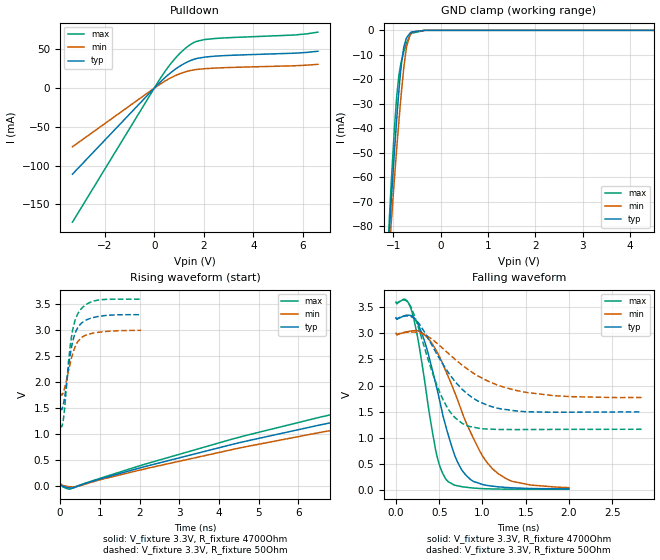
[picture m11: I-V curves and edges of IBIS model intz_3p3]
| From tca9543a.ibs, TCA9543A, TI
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|   intz_3p3 Model
[Model]   intz_3p3
Model_type   Open_drain
Polarity   Non-Inverting
Vmeas = 1.65
Vref = 3.3
Cref = 100pF
Rref = 4700
|   typ   min   max
|   (nom PVT)   (fast PVT)   (slow PVT)
C_comp   1.585e-12   1.479e-12   1.813e-12
| Where nom  PVT is Nominal Process, 3.3V, 27C
|   Fast PVT is Strong Process,  3.6V, -40C
|   Slow PVT is Weak Process,   3V, 85C
[Voltage Range]   3.3   3   3.6
|Junction Temperature
[Temperature Range]   27   85   -40
[Pullup Reference]   3.3   3   3.6
[Pulldown Reference]   0   0   0
[Power Clamp Reference]   3.3   3   3.6
[GND Clamp Reference]   0   0   0
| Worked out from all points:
|   slope of the pulldown table from 0 to 0.495 V, typ, clamps not added: 32.1 ohm
|   GND clamp passes 1 mA (typ) near -0.64 V on its own axis
|   falling waveform, V_fixture 3.3V, R_fixture 4700Ohm: 20-80 % time 309ps typ, 464ps min, 208ps max; typ from 3.3 V to 0.019 V
|   rising waveform, V_fixture 3.3V, R_fixture 4700Ohm: 20-80 % time 18ns typ, 18.9ns min, 17.1ns max; typ from 0.02 V to 3.3 V
|   falling waveform, V_fixture 3.3V, R_fixture 50Ohm: 20-80 % time 455ps typ, 651ps min, 310ps max; typ from 3.3 V to 1.5 V
|   rising waveform, V_fixture 3.3V, R_fixture 50Ohm: 20-80 % time 237ps typ, 266ps min, 218ps max; typ from 1.5 V to 3.3 V
[Pulldown]
|   Voltage   I(typ)   I(min)   I(max)
-3.3V     -111mA     -75.61mA   -172.9mA
243mV     7.977mA    5.352mA    12.58mA
558mV     17.19mA    11.45mA    27.09mA
843.6mV   24.36mA    16.07mA    38.41mA
1.32V     33.59mA    21.66mA    53.11mA
1.647V    37.69mA    23.83mA    59.61mA
2.052V    40.16mA    25.17mA    62.81mA
3.231V    42.56mA    26.86mA    65.44mA
5.642V    45.12mA    28.87mA    68.56mA
6.6V      47.62mA    30.78mA    72.34mA
[GND Clamp]
|   Voltage   I(typ)   I(min)   I(max)
-3.3V     -900.9mA   -814.7mA   -1.047A
-1.169V   -109.9mA   -114.6mA   -110.1mA
-1.047V   -71.3mA    -80.31mA   -64.43mA
-974.4mV  -49.75mA   -60.85mA   -40.2mA
-924mV    -35.82mA   -47.94mA   -26.61mA
-880.8mV  -24.97mA   -37.42mA   -18.62mA
-823.2mV  -13.15mA   -24.49mA   -12.34mA
-775.5mV  -6.819mA   -15.22mA   -8.668mA
-717mV    -3.044mA   -6.672mA   -5.061mA
-612mV    -674.2uA   -730.5uA   -1.179mA
-330mV    -1.399uA   -1.345uA   -1.097uA
6.6V      0A         0A         0A
[POWER Clamp]
|   Voltage   I(typ)   I(min)   I(max)
-3.3V     0A         0A         0A
-3.243V   0A         0A         0A
6.6V      0A         0A         0A
[Ramp]
R_load = 4700
|   typ   min   max
dV/dt_r   1.96775/1.80168e-08   1.7835/1.8882e-08   2.15152/1.71709e-08
dV/dt_f   1.96775/3.0818e-10   1.7835/4.67542e-10   2.15152/2.07559e-10
[Falling Waveform]
V_fixture = 3.3V
V_fixture_min = 3V
V_fixture_max = 3.6V
R_fixture = 4700Ohm
|   Time   V(typ)   V(min)   V(max)
0s        3.3V       3V         3.6V
110ps     3.345V     3.024V     3.65V
190ps     3.329V     3.049V     3.383V
320ps     2.904V     2.987V     2.218V
460ps     2.036V     2.69V      750.4mV
590ps     1.137V     2.226V     179.2mV
790ps     317.7mV    1.373V     53.4mV
1.12ns    69.76mV    397.3mV    16.29mV
1.35ns    37.45mV    160.9mV    12.52mV
2ns       18.86mV    41.74mV    14mV
[Rising Waveform]
V_fixture = 3.3V
V_fixture_min = 3V
V_fixture_max = 3.6V
R_fixture = 4700Ohm
|   Time   V(typ)   V(min)   V(max)
0s        20.41mV    27.49mV    14.13mV
260ps     -38.28mV   -16.59mV   -57.82mV
2.12ns    371.6mV    327.3mV    417mV
6.54ns    1.176V     1.032V     1.325V
11.63ns   1.854V     1.634V     2.08V
18.73ns   2.471V     2.193V     2.753V
26.18ns   2.85V      2.545V     3.159V
35.29ns   3.098V     2.787V     3.419V
48.28ns   3.249V     2.94V      3.561V
99.99ns   3.3V       3V         3.6V
[Falling Waveform]
V_fixture = 3.3V
V_fixture_min = 3V
V_fixture_max = 3.6V
R_fixture = 50Ohm
|   Time   V(typ)   V(min)   V(max)
0s        3.3V       3V         3.6V
100ps     3.331V     3.019V     3.639V
170ps     3.326V     3.026V     3.515V
270ps     3.18V      3.014V     3.054V
540ps     2.417V     2.716V     1.744V
660ps     2.127V     2.536V     1.424V
810ps     1.862V     2.335V     1.237V
1.09ns    1.605V     2.067V     1.164V
1.51ns    1.497V     1.867V     1.156V
2.84ns    1.495V     1.771V     1.161V
[Rising Waveform]
V_fixture = 3.3V
V_fixture_min = 3V
V_fixture_max = 3.6V
R_fixture = 50Ohm
|   Time   V(typ)   V(min)   V(max)
0s        1.497V     1.781V     1.16V
40ps      1.475V     1.751V     1.148V
90ps      1.607V     1.826V     1.338V
210ps     2.28V      2.213V     2.393V
290ps     2.687V     2.48V      2.897V
370ps     2.925V     2.672V     3.177V
470ps     3.078V     2.807V     3.353V
650ps     3.197V     2.907V     3.497V
910ps     3.261V     2.957V     3.576V
2.04ns    3.302V     3.001V     3.6V
